FUNCTION FC 9 : VOID
TITLE =COMANDI PROFIBUS AZIONAMENTO 9 PROFILA 7 (SLAVE 6)
VERSION : 0.1

BEGIN
NETWORK
TITLE =TRASFERISCO I SEGNALI DI COMANDO
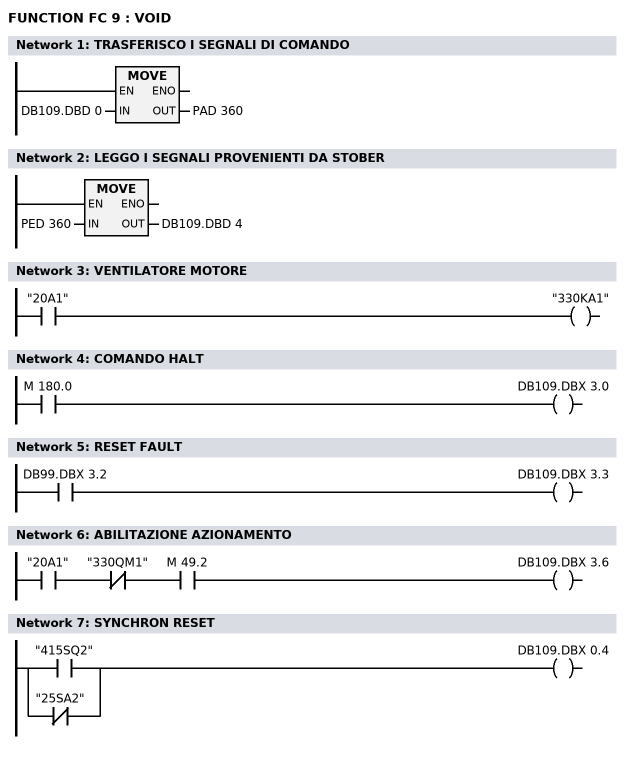
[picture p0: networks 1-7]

      L     DB109.DBD    0;
      T     PAD  360;
      NOP   0;
NETWORK
TITLE =LEGGO I SEGNALI PROVENIENTI DA STOBER

      L     PED  360;
      T     DB109.DBD    4;
      NOP   0;
NETWORK
TITLE =VENTILATORE MOTORE

      U     "20A1";
      =     "330KA1";
NETWORK
TITLE =COMANDO HALT

      U     M    180.0;
      =     DB109.DBX    3.0;
NETWORK
TITLE =RESET FAULT

      U     DB99.DBX    3.2;
      =     DB109.DBX    3.3;
NETWORK
TITLE =ABILITAZIONE AZIONAMENTO

      U     "20A1";
      UN    "330QM1";
      U     M     49.2;
      =     DB109.DBX    3.6;
NETWORK
TITLE =SYNCHRON RESET

      O     "415SQ2";
      ON    "25SA2";
      =     DB109.DBX    0.4;
END_FUNCTION

